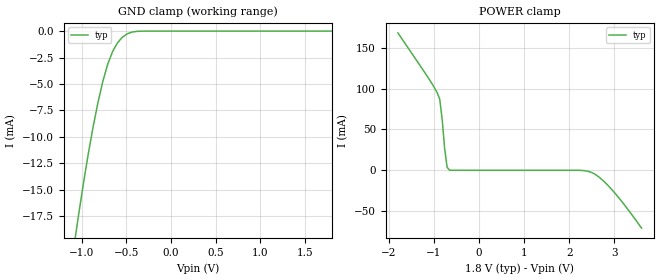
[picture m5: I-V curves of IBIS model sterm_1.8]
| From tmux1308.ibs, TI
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| sterm_1.8
[Model]   sterm_1.8
Model_type   Terminator
|   typ   min   max
C_comp   6.362683e-13   NA   NA
[Voltage Range]   1.8   NA   NA
[Temperature Range]   27   NA   NA
[Power Clamp Reference]   1.8   NA   NA
[GND Clamp Reference]   0   NA   NA
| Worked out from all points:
|   GND clamp passes 1 mA (typ) near -0.59 V on its own axis
|   POWER clamp passes 1 mA (typ) near -0.67 V on its own axis
[GND Clamp]
|   Voltage   I(typ)   I(min)   I(max)
-3.6V     -4.477kA   NA         NA
-1.091V   -20.63mA   NA         NA
-1.036V   -17.46mA   NA         NA
-927.3mV  -11.66mA   NA         NA
-872.7mV  -9.074mA   NA         NA
-763.6mV  -4.757mA   NA         NA
-709.1mV  -3.138mA   NA         NA
-654.5mV  -1.938mA   NA         NA
-545.5mV  -582.8uA   NA         NA
-436.4mV  -95.88uA   NA         NA
-327.3mV  -6.698uA   NA         NA
1.8V      873.5pA    NA         NA
[POWER Clamp]
|   Voltage   I(typ)   I(min)   I(max)
-1.8V     168.2mA    NA         NA
-1.091V   110.1mA    NA         NA
-927.3mV  94.67mA    NA         NA
-872.7mV  87.09mA    NA         NA
-818.2mV  62.25mA    NA         NA
-763.6mV  26.55mA    NA         NA
-709.1mV  3.607mA    NA         NA
-654.5mV  97.04uA    NA         NA
2.455V    -1.938mA   NA         NA
2.673V    -9.074mA   NA         NA
2.891V    -20.63mA   NA         NA
3.6V      -70.89mA   NA         NA
